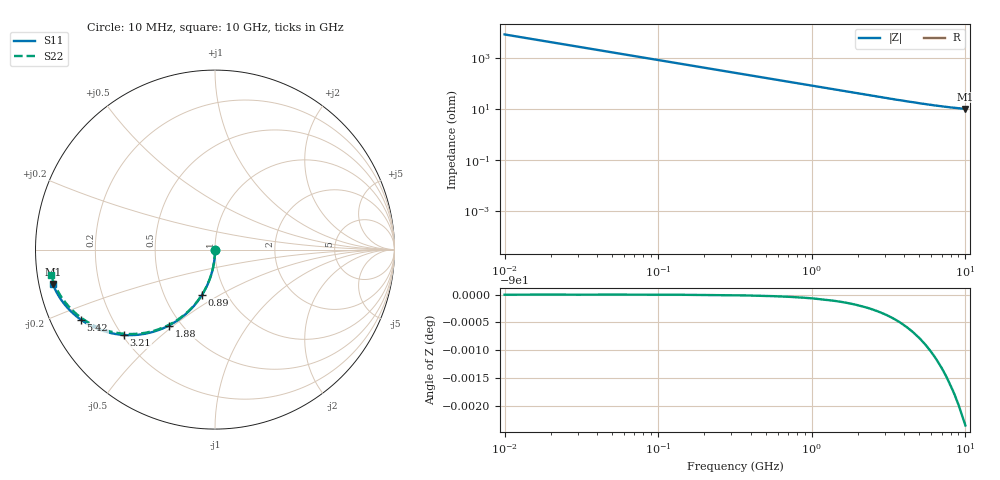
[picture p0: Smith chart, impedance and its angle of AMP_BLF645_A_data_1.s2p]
! Created Mon Mar 08 12:01:49 2010
# ghz S ma R 50
! 2 Port Network Data from SP1.SP block
! freq  magS11  angS11  magS21  angS21  magS12  angS12  magS22  angS22
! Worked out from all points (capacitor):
!   1000 points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, 10 MHz to 10 GHz, reference 50 ohm
!   read as one part in shunt: C = 1.98 pF near 60 MHz
!   lowest |Z| = 10 ohm at 10 GHz (marker M1)
!   S11 on the Smith chart (normalised r, x): 10 MHz: 1.00, -0.01; 890 MHz: 0.77, -0.41; 1.88 GHz: 0.43, -0.48; 3.21 GHz: 0.21, -0.38; 5.42 GHz: 0.09, -0.24; 10 GHz: 0.04, -0.10
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0.01  0.003026 -90.2  1 -0.2  1 -0.2  0.003026 -90.2
0.04  0.0121 -90.7  0.9999 -0.7  0.9999 -0.7  0.0121 -90.7
0.07  0.02118 -91.3  0.9998 -1.3  0.9998 -1.3  0.02118 -91.3
0.1  0.03025 -91.8  0.9995 -1.8  0.9995 -1.8  0.03025 -91.8
0.15  0.04535 -92.7  0.999 -2.7  0.999 -2.7  0.04535 -92.8
0.23  0.06946 -94.2  0.9976 -4.2  0.9976 -4.2  0.06946 -94.2
0.34  0.1024 -96.2  0.9947 -6.2  0.9947 -6.2  0.1024 -96.2
0.49  0.1469 -98.8  0.9892 -8.9  0.9892 -8.9  0.1469 -99.0
0.67  0.1991 -102.0  0.98 -12.1  0.98 -12.1  0.1991 -102.2
0.89  0.2607 -105.8  0.9654 -16.0  0.9654 -16.0  0.2607 -106.1
1.25  0.3548 -111.8  0.9349 -22.0  0.9349 -22.0  0.3548 -112.1
1.68  0.4544 -118.4  0.8908 -28.7  0.8908 -28.7  0.4544 -118.9
1.88  0.4956 -121.3  0.8685 -31.5  0.8685 -31.5  0.4956 -121.8
2.49  0.6019 -129.1  0.7986 -39.5  0.7986 -39.5  0.6019 -129.8
3.21  0.6946 -136.8  0.7194 -47.2  0.7194 -47.2  0.6946 -137.6
3.34  0.7082 -138.0  0.706 -48.4  0.706 -48.4  0.7082 -138.9
4.14  0.7757 -144.5  0.6311 -55.1  0.6311 -55.1  0.7757 -145.6
5.01  0.8254 -150.1  0.5645 -60.8  0.5645 -60.8  0.8254 -151.5
5.42  0.8429 -152.4  0.5381 -63.1  0.5381 -63.1  0.8429 -153.9
6.67  0.8807 -158.0  0.4736 -69.0  0.4736 -69.0  0.8807 -159.9
8.34  0.9092 -163.7  0.4163 -74.9  0.4163 -74.9  0.9092 -166.1
10  0.9241 -168.1  0.3821 -79.6  0.3821 -79.6  0.9241 -171.2
